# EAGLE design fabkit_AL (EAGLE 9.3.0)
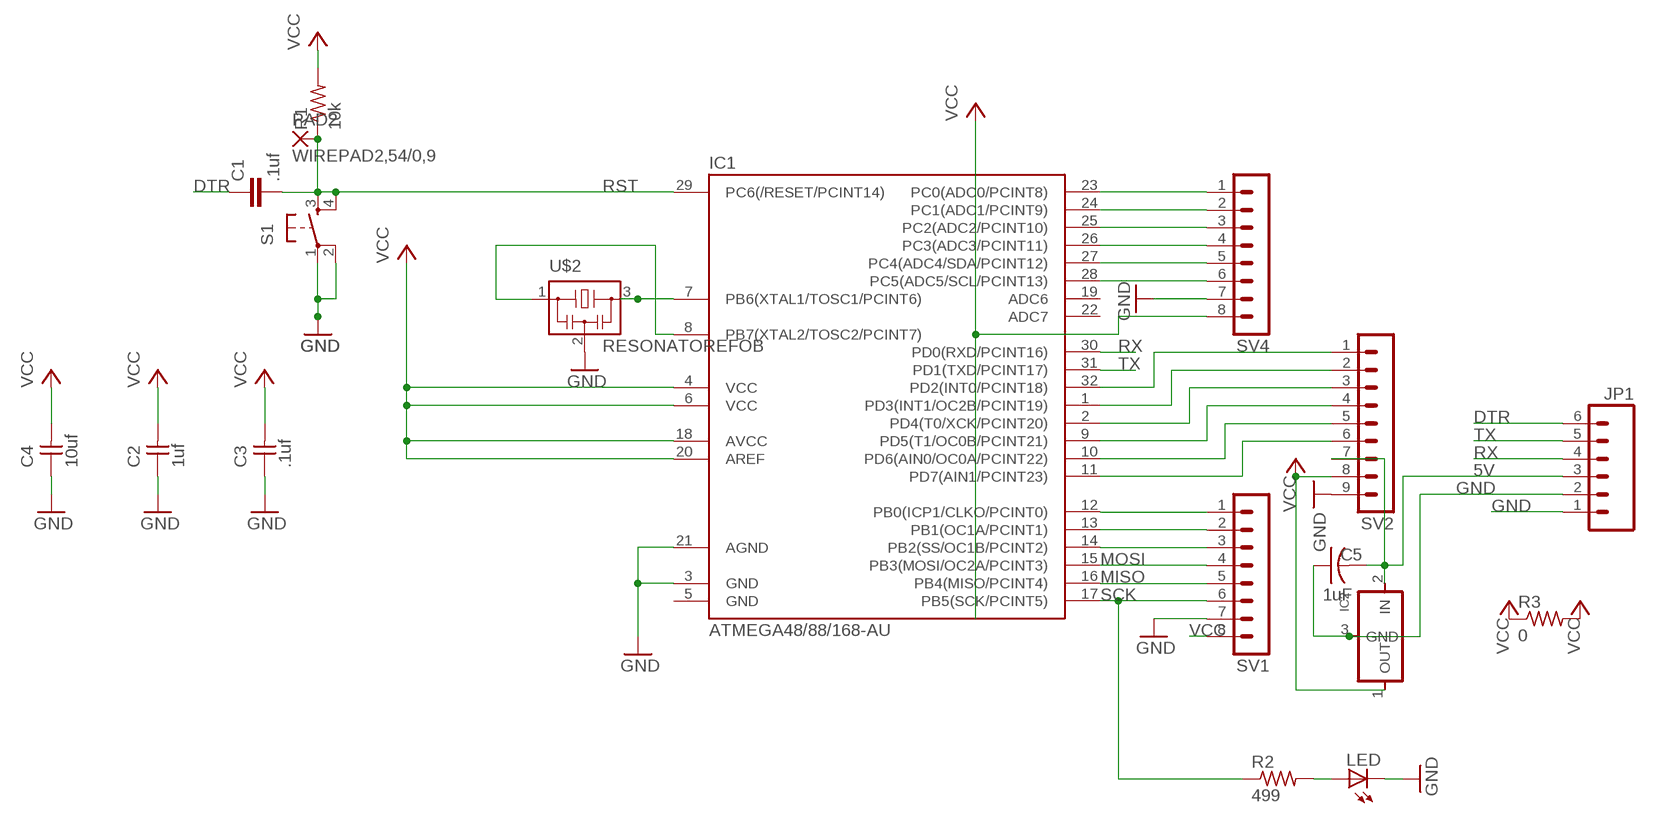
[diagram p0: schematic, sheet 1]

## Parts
C1  .1uf  C-EUC1206  [C1206]
C2  1uf  UNPOLARIZED_CAPACITOR1206  [1206]
C3  .1uf  UNPOLARIZED_CAPACITOR1206  [1206]
C4  10uf  UNPOLARIZED_CAPACITOR1206  [1206]
C5  1uF  CAP-US1206FAB  [C1206FAB]
IC1  ATMEGA48/88/168-AU  [TQFP32-08]
IC2  REGULATORSOT23  [SOT23]
JP1  M06SMD  [1X06-SMD]
LED  LED1206  [1206]
PAD2  WIREPAD2,54/0,9  [2,54/0,9]
R1  10k  RESISTOR1206  [1206]
R2  499  RESISTOR1206  [1206]
R3  0  RES-US1206FAB  [R1206FAB]
S1  6MM_SWITCH6MM_SWITCH  [6MM_SWITCH]
SV1  MA08-1  [MA08-1]
SV2  MA09-1  [MA09-1]
SV4  MA08-1  [MA08-1]
U$2  RESONATOREFOB  [EFOBM]

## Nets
5V: C5.2 IC2.2(IN) JP1.3 SV2.7
DTR: C1.1 JP1.6
GND: C2.1 C3.1 C4.1 C5.1 IC1.3(GND) IC1.21(AGND) IC2.3(GND) JP1.1 JP1.2 LED.2(C) S1.1(P) S1.2(P1) SV1.7 SV2.9 SV4.7 U$2.2
MISO: IC1.16(PB4(MISO/PCINT4)) SV1.5
MOSI: IC1.15(PB3(MOSI/OC2A/PCINT3)) SV1.4
N$1: IC1.8(PB7(XTAL2/TOSC2/PCINT7)) U$2.1
N$2: IC1.12(PB0(ICP1/CLKO/PCINT0)) SV1.1
N$3: IC1.23(PC0(ADC0/PCINT8)) SV4.1
N$4: IC1.24(PC1(ADC1/PCINT9)) SV4.2
N$5: IC1.25(PC2(ADC2/PCINT10)) SV4.3
N$6: IC1.26(PC3(ADC3/PCINT11)) SV4.4
N$7: IC1.27(PC4(ADC4/SDA/PCINT12)) SV4.5
N$8: IC1.28(PC5(ADC5/SCL/PCINT13)) SV4.6
N$9: IC1.7(PB6(XTAL1/TOSC1/PCINT6)) U$2.3
N$10: IC1.32(PD2(INT0/PCINT18)) SV2.1
N$11: IC1.1(PD3(INT1/OC2B/PCINT19)) SV2.2
N$12: IC1.2(PD4(T0/XCK/PCINT20)) SV2.3
N$13: IC1.9(PD5(T1/OC0B/PCINT21)) SV2.4
N$14: IC1.10(PD6(AIN0/OC0A/PCINT22)) SV2.5
N$15: IC1.11(PD7(AIN1/PCINT23)) SV2.6
N$17: IC1.13(PB1(OC1A/PCINT1)) SV1.2
N$18: IC1.14(PB2(SS/OC1B/PCINT2)) SV1.3
N$23: LED.1(A) R2.2
RST: C1.2 IC1.29(PC6(/RESET/PCINT14)) PAD2.1(P) R1.1 S1.3(S) S1.4(S1)
RX: IC1.30(PD0(RXD/PCINT16)) JP1.4
SCK: IC1.17(PB5(SCK/PCINT5)) R2.1 SV1.6
TX: IC1.31(PD1(TXD/PCINT17)) JP1.5
VCC: C2.2 C3.2 C4.2 IC1.4(VCC) IC1.6(VCC) IC1.18(AVCC) IC1.20(AREF) IC2.1(OUT) R1.2 R3.1 R3.2 SV1.8 SV2.8 SV4.8
Unconnected: IC1.19(ADC6) IC1.22(ADC7)

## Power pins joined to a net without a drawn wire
GND: IC1.5(GND)

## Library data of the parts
C1 = rcl:C-EU: CAPACITOR, European symbol
C2-C4 = ng:UNPOLARIZED_CAPACITOR: unpolarized_capacitor
C5 = fab:CAP-US
IC1 = atmega8:ATMEGA48/88/168
IC2 = fab:REGULATOR
JP1 = SparkFun:M06: Header 6 Standard 6-pin 0.1" header. Use with straight break away headers (SKU : PRT-00116), right angle break away headers (PRT-00553), swiss pins (PRT-00743), machine pins (PRT-00117), and female headers (PRT-00115). Molex polarized connector foot print use with SKU : PRT-08094 with associated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
LED = ng:LED
PAD2 = wirepad:WIREPAD: Wire PAD connect wire on PCB
R1 R2 = ng:RESISTOR
R3 = fab:RES-US: Resistor (US Symbol)
S1 = ng:6MM_SWITCH: OMRON SWITCH
SV1 SV4 = con-lstb:MA08-1: PIN HEADER
SV2 = con-lstb:MA09-1: PIN HEADER; OC_FARNELL: unknown; OC_NEWARK: unknown
U$2 = fab:RESONATOR

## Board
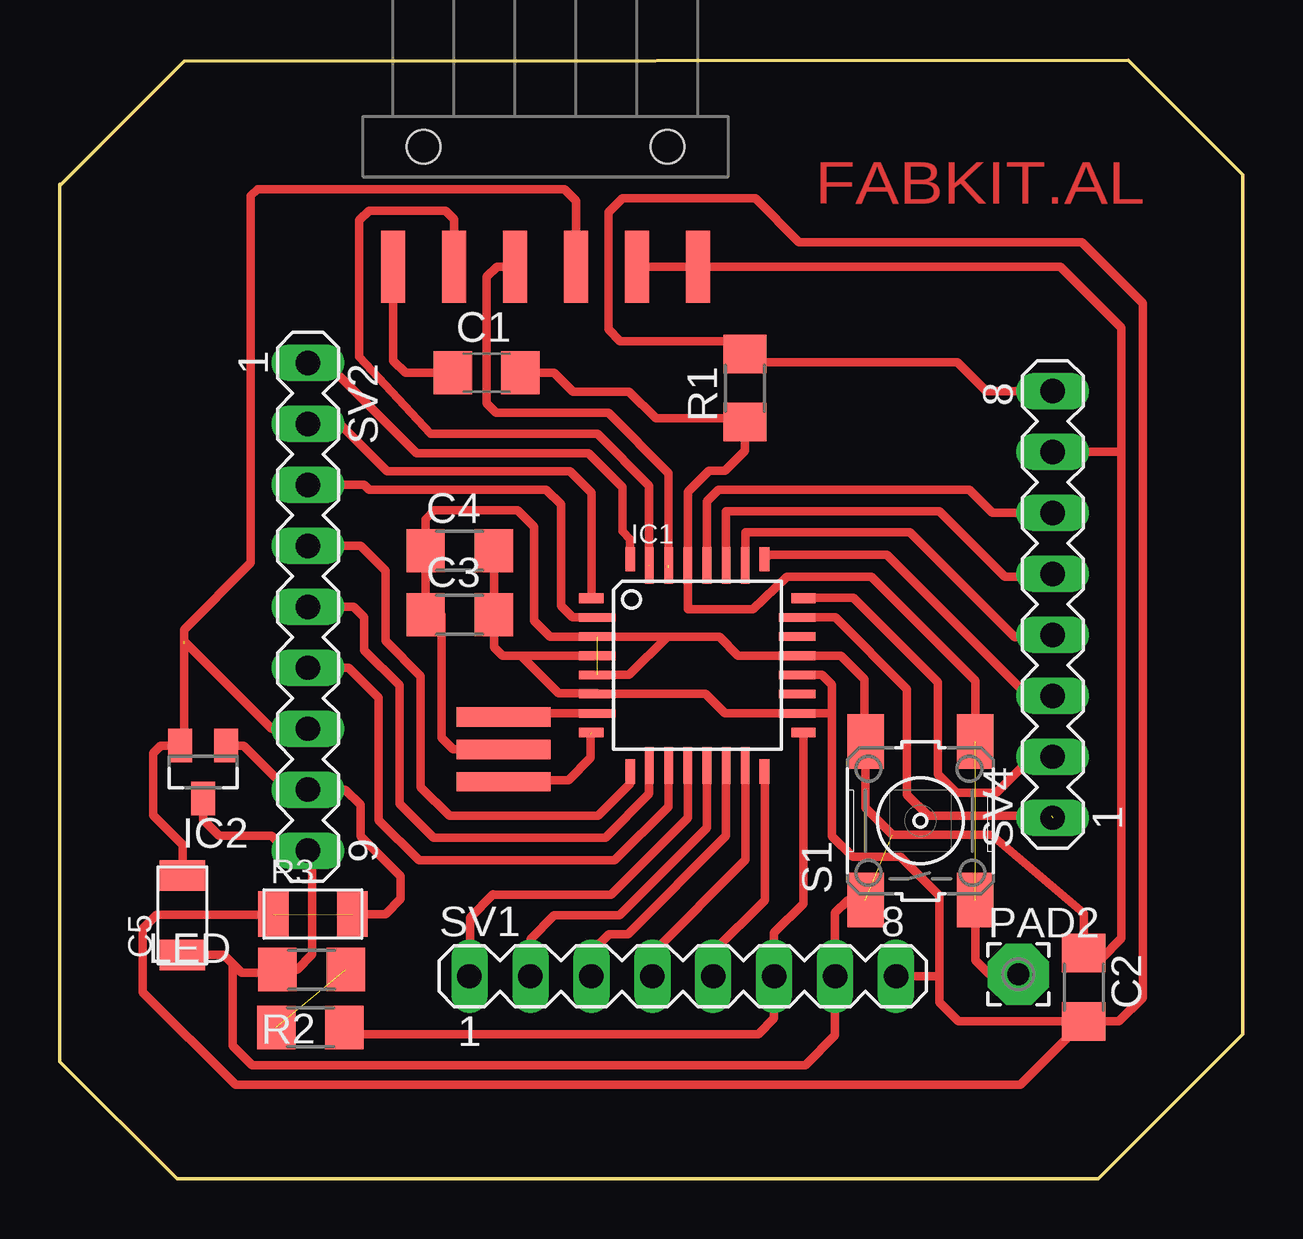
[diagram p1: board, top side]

Size 49.3 x 46.61 mm. Coordinates in mm from the lower left corner, seen from the top.
Outline: 0,41.38 5.18,46.56 44.53,46.61 49.3,41.83 49.3,6.02 43.28,0 4.88,0 0,4.88 0,41.43
Copper layers (1*16): Top 0.035mm / dielectric 1.5mm / Bottom 0.035mm
Design rules "default *": minimum track width 10mil, minimum drill 24mil, track to track 16mil, track to pad 16mil, pad to pad 16mil, via to via 16mil, smd to smd 16mil, copper to edge 16mil, drill to drill 8mil, minimum pad ring 10mil, minimum via ring 8mil, stop-mask expansion 4mil, vias tented up to drill 0mil, thermal gap 10mil

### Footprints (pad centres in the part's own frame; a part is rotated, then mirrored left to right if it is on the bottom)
C1206 = smd 1.6 x 1.8: 1 -1.4,0; 2 1.4,0
1206 = smd 1.6 x 1.803: 1 -1.422,0; 2 1.422,0
C1206FAB = smd 1.27 x 1.905: 1 -1.651,0; 2 1.651,0
TQFP32-08 = smd 1.016 x 0.406: 1 -4.42,2.8; 8 -4.42,-2.8; 17 4.42,-2.8; 24 4.42,2.8 | smd 1.524 x 0.356: 2 -4.166,2; 3 -4.166,1.2; 4 -4.166,0.4; 5 -4.166,-0.4; 6 -4.166,-1.2; 7 -4.166,-2; 18 4.166,-2; 19 4.166,-1.2; 20 4.166,-0.4; 21 4.166,0.4; 22 4.166,1.2; 23 4.166,2 | smd 0.406 x 1.016: 9 -2.8,-4.42; 16 2.8,-4.42; 25 2.8,4.42; 32 -2.8,4.42 | smd 0.356 x 1.524: 10 -2,-4.166; 11 -1.2,-4.166; 12 -0.4,-4.166; 13 0.4,-4.166; 14 1.2,-4.166; 15 2,-4.166; 26 2,4.166; 27 1.2,4.166; 28 0.4,4.166; 29 -0.4,4.166; 30 -1.2,4.166; 31 -2,4.166
SOT23 = smd 1 x 1.4: 1 -0.95,-1.1; 2 0.95,-1.1; 3 0,1.1
1X06-SMD = smd 1 x 3: 1 -6.35,5; 2 -3.81,5; 3 -1.27,5; 4 1.27,5; 5 3.81,5; 6 6.35,5 | hole 1.4: -5.08,0; 5.08,0
2,54/0,9 = drill 0.914 pad 2.54 octagon: 1 0,0
R1206FAB = smd 1.27 x 1.905: 1 -1.651,0; 2 1.651,0
6MM_SWITCH = smd 2.286 x 1.524: 1 -3.302,2.286; 2 3.302,2.286; 3 -3.302,-2.286; 4 3.302,-2.286
MA08-1 = drill 1.016 long: 1 -8.89,0; 2 -6.35,0; 3 -3.81,0; 4 -1.27,0; 5 1.27,0; 6 3.81,0; 7 6.35,0; 8 8.89,0
MA09-1 = drill 1.016 long: 1 -10.16,0; 2 -7.62,0; 3 -5.08,0; 4 -2.54,0; 5 0,0; 6 2.54,0; 7 5.08,0; 8 7.62,0; 9 10.16,0
EFOBM = smd 0.8 x 3.9: 1 -1.35,0; 2 0,0; 3 1.35,0

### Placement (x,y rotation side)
C1  17.78,33.58 0 top
C2  42.67,7.98 270 top
C3  16.66,23.49 0 top
C4  16.66,26.16 0 top
C5  5.11,10.97 90 top
IC1  26.57,21.39 0 top
IC2  5.97,16.94 180 top
JP1  20.24,43 180 top
LED  10.49,8.71 180 top
PAD2  39.95,8.51 0 top
R1  28.55,32.94 90 top
R2  10.44,6.3 180 top
R3  10.54,11.02 0 top
S1  35.86,14.91 90 top
SV1  25.96,8.43 0 top
SV2  10.34,23.83 270 top
SV4  41.38,23.93 90 top
U$2  18.49,17.88 90 top

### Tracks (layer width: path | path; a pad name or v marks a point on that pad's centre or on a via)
5V  (1 unrouted)
  Top 0.356: JP1.3 21.51,40.74 21.03,41.22 8.23,41.22 7.95,40.94 7.95,25.65 5.17,22.87 5.17,22.39 8.81,18.74 SV2.7 | 5.17,22.28 5.17,18.19 IC2.2 | IC2.2 4.99,18.07 | C5.2 5.11,13.92 3.89,15.14 3.89,17.73 4.2,18.04 IC2.2
DTR
  Top 0.356: JP1.6 13.89,34.09 14.4,33.58 C1.1
GND  (2 unrouted)
  Top 0.356: 30.63,21.79 IC1.21 | IC1.21 32.54,21.79 33.53,20.8 33.53,17.63 S1.2 33.58,15.44 34.7,14.33 38.83,14.33 42.67,11.05 C2.1 42.57,9.17 43.41,9.17 44.25,10.01 44.25,30.28 | JP1.2 JP1.1 41.71,38 44.25,35.46 44.25,30.28 | 25.32,22.58 27.48,22.58 28.27,21.79 IC1.21 | IC1.5 23.72,20.99 25.32,22.58 | 44.25,30.28 SV4.7 41.33,30.23 | C4.1 15.27,26.19 | C4.1 C3.1 15.9,23.49 15.9,18.36 16.38,17.88 U$2.2 | C4.1 15.24,27.48 15.6,27.84 19.08,27.84 19.76,27.15 19.76,23.25 20.43,22.58 25.32,22.58 | 7.19,8.92 7.19,5.54 8,4.72 31.06,4.72 32.31,5.97 SV1.7 32.31,11.07 32.84,11.61 S1.1 | C5.1 6.83,9.32 7.57,8.58 8.94,8.58 LED.2 9.88,8.71 10.52,9.35 10.52,13.49 SV2.9 9.45,13.66 8.82,14.29 6.63,14.29 5.97,14.95 IC2.3
MISO
  Top 0.356: SV1.5 27.23,9.45 29.39,11.61 29.39,16.95 IC1.16
MOSI
  Top 0.356: SV1.4 24.69,9.4 28.58,13.28 IC1.15
N$1  (1 unrouted)
  Top 0.356: 22.12,18.48 22.12,17.53 21.21,16.61 18.49,16.61 U$2.1
N$2
  Top 0.356: SV1.1 17.09,10.87 18.06,11.84 22.96,11.84 26.17,15.04 IC1.12
N$3  (1 unrouted)
  Top 0.356: IC1.23 32.32,23.39 35.31,20.4 35.31,16 36.2,15.11 41.33,15.11
N$4
  Top 0.356: 30.94,24.18 30.94,24.19 IC1.24 31.01,24.21 33.07,24.21 36.6,20.68 36.6,16.84 37.36,16.08 39.04,16.08 40.54,17.58 SV4.2
N$5
  Top 0.356: IC1.25 29.55,25.98 34.47,25.98 40.36,20.09 41.35,20.09 SV4.3
N$6
  Top 0.356: IC1.26 28.57,26.92 35.43,26.92 39.8,22.55 41.28,22.55 SV4.4
N$7
  Top 0.356: IC1.27 27.77,27.81 36.65,27.81 39.4,25.07 41.25,25.07 SV4.5
N$8
  Top 0.356: SV4.6 38.86,27.74 37.9,28.7 27.45,28.7 26.97,28.22 IC1.28
N$9
  Top 0.356: IC1.7 18.65,19.39 arc90 U$2.3
N$10
  Top 0.356: IC1.32 23.77,26.64 23.44,26.97 23.44,28.81 22.02,30.23 14.86,30.23 11.1,33.98 SV2.1
N$11
  Top 0.356: IC1.1 22.15,28.57 21.26,29.46 13.64,29.46 11.66,31.44 SV2.2
N$12
  Top 0.356: IC1.2 21.36,23.39 20.88,23.87 20.88,28.09 20.27,28.7 12.88,28.7 12.67,28.9 SV2.3
N$13
  Top 0.356: 23.77,16.76 IC1.9 23.77,16.46 22.42,15.11 16.23,15.11 15.04,16.31 15.04,20.93 13.56,22.4 13.56,25.32 12.52,26.36 SV2.4
N$14
  Top 0.356: IC1.10 24.56,17.14 24.56,16.03 22.73,14.2 15.57,14.2 14.15,15.62 14.15,20.55 12.67,22.02 12.67,23.39 12.24,23.82 SV2.5
N$15
  Top 0.356: IC1.11 25.37,15.49 23.11,13.26 14.96,13.26 13.28,14.93 13.28,20.04 12.04,21.28 SV2.6
N$17
  Top 0.356: IC1.13 26.97,14.62 23.32,10.97 20.6,10.97 19.61,9.98 SV1.2
N$18
  Top 0.356: IC1.14 27.77,14.28 23.67,10.19 22.89,10.19 22.15,9.45 SV1.3
N$23  (1 unrouted)
RST  (1 unrouted)
  Top 0.356: C1.2 20.6,33.58 21.39,32.79 23.72,32.79 24.84,31.67 28.4,31.67 R1.1 28.55,30.33 27.71,29.5 27.05,29.5 26.17,28.61 IC1.29 26.17,23.72 28.88,23.72 30.3,25.07 33.83,25.07 38.15,20.75 S1.4 | S1.3 38.15,9.09 38.74,8.51 PAD2.1
RX  (1 unrouted)
  Top 0.356: 25.37,25.45 25.37,29.39 22.86,31.9 18.19,31.9 17.78,32.31 17.78,37.57 18.21,38 JP1.4
SCK
  Top 0.356: IC1.17 30.99,11.46 29.77,10.24 SV1.6 29.77,6.68 29.11,6.02 12.14,6.02 R2.1
TX  (1 unrouted)
  Top 0.356: JP1.5 16.43,39.98 16.08,40.33 12.88,40.33 12.47,39.93 12.47,34.24 15.45,31.04 22.4,31.04 24.56,28.88 IC1.31
VCC  (2 unrouted)
  Top 0.356: 27.94,34.29 28.07,34.32 | 27.91,34.32 27.94,34.29 | R1.2 28.91,34.01 37.41,34.01 38.61,32.82 SV4.8 | 42.75,6.71 C2.2 | IC1.6 | 32.18,19.39 32.18,20.57 31.77,20.99 IC1.20 | 32.18,19.39 32.18,14.27 33.05,13.41 35.03,13.41 36.65,11.79 36.65,8.43 | 32.18,19.39 IC1.18 27.71,19.38 26.9,20.19 IC1.6 | 27.94,34.29 28.09,34.16 R1.2 | C4.2 C3.2 18.09,22.15 18.45,21.79 19.21,21.79 | C2.2 44.15,6.55 45.14,7.54 45.14,36.47 42.6,39.01 30.81,39.01 28.98,40.84 23.44,40.84 22.86,40.26 22.86,35.38 23.34,34.9 28.02,34.9 R1.2 | 36.65,8.43 36.65,7.34 37.44,6.55 C2.2 | SV1.8 36.65,8.43 | IC1.4 19.21,21.79 | 19.21,21.79 20.78,20.22 22.38,20.22 IC1.6 | C2.2 40.03,3.91 7.32,3.91 3.45,7.77 3.45,10.41 4.04,11 8.99,11 | IC2.1 7.66,18.04 9.5,16.2 SV2.8 11.89,16.2 12.52,15.57 12.52,14.27 14.2,12.6 14.2,11.66 13.56,11.02 R3.2

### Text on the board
Top: FABKIT.AL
